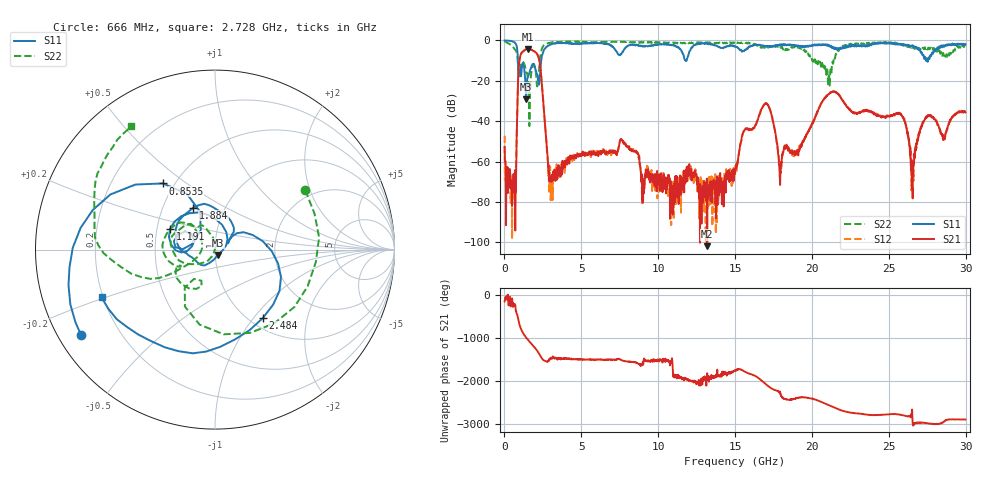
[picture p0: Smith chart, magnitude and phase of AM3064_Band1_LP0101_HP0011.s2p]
# Hz S DB R 50.0
!freq dBS11 angS11 dBS21 angS21 dBS12 angS12 dBS22 angS22
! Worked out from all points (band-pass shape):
!   1600 points, 10 MHz to 29.98 GHz, reference 50 ohm
!   highest |S21| = -4.21 dB at 1.528 GHz (marker M1); lowest = -101.9 dB at 13.19 GHz (marker M2)
!   |S21| within 3 dB of the highest: 1.051 GHz to 2.155 GHz (1.105 GHz wide, 68.9 % of centre)
!   lowest |S11| = -29.2 dB at 1.416 GHz (marker M3), VSWR 1.07, Z = 51.7 - j3.07 ohm
!   |S11| at or under -10 dB: 876.5 MHz to 2.391 GHz (1.514 GHz wide, 92.7 % of centre); 11.78 GHz to 11.84 GHz (66.4 MHz wide, 0.562 % of centre); 27.41267 GHz to 27.43596 GHz (23.29 MHz wide, 0.0849 % of centre)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
!   |S22| runs from -42.4 to -0.4 dB; largest |S21 - S12| = 0.0081
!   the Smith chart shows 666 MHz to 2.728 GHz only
!   S11 on the Smith chart (normalised r, x): 666 MHz: 0.07, -0.29; 853.5 MHz: 0.43, +0.41; 1.191 GHz: 0.59, +0.15; 1.884 GHz: 0.71, +0.36; 2.484 GHz: 1.14, -1.12; 2.728 GHz: 0.19, -0.20
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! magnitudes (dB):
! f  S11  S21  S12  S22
! 10 MHz  0.0  -52.7  -47.2  -0.4
! 666 MHz  -1.1  -71.3  -73.4  -4.4
! 853.5 MHz  -6.6  -28.0  -27.9  -8.9
! 1.191 GHz  -11.2  -5.6  -5.6  -10.7
! 1.416 GHz  -29.2  -4.3  -4.3  -16.0
! 1.528 GHz  -18.2  -4.2  -4.2  -19.3
! 1.884 GHz  -11.6  -5.2  -5.2  -11.9
! 2.484 GHz  -6.6  -26.3  -26.2  -3.3
! 2.728 GHz  -3.3  -50.2  -50.7  -1.6
! 3.046 GHz  -1.9  -70.0  -69.9  -1.0
! 5.015 GHz  -1.5  -57.2  -57.2  -0.7
! 10 GHz  -2.0  -69.6  -66.9  -1.0
! 13.19 GHz  -1.4  -101.9  -80.1  -1.1
! 15 GHz  -3.0  -66.1  -64.0  -1.4
! 16.94 GHz  -2.7  -31.5  -31.4  -3.6
! 17.95 GHz  -2.3  -64.9  -66.0  -3.1
! 19.99 GHz  -2.8  -41.5  -41.4  -9.3
! 21.36 GHz  -3.2  -25.4  -25.2  -11.4
! 25 GHz  -1.1  -37.4  -37.5  -1.2
! 26.53 GHz  -2.4  -73.2  -62.8  -4.2
! 27.43 GHz  -10.1  -37.9  -37.7  -3.9
! 29.98 GHz  -1.9  -35.7  -35.6  -2.8
